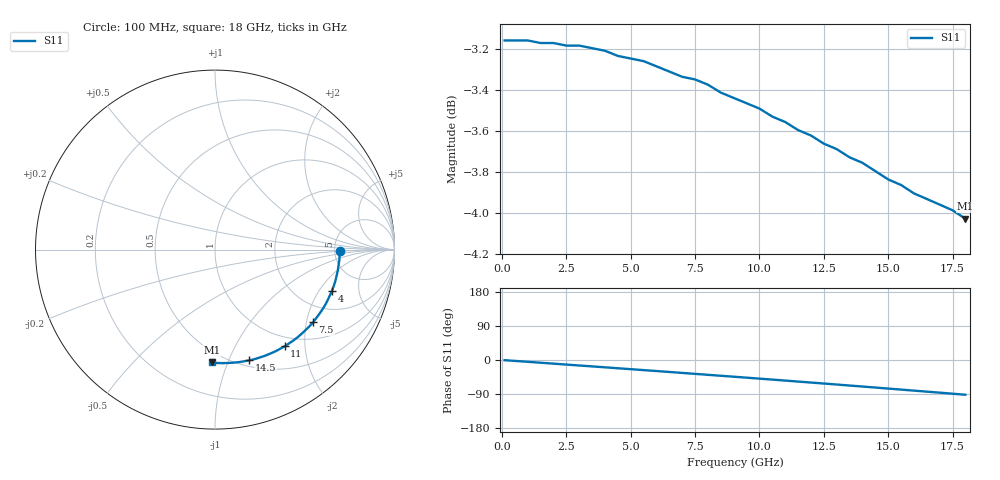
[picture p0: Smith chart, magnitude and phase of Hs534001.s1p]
!HSCH-5320 and HSCH-5340 Schottky diodes
!S-parameters at 1 mA self-bias.  Last updated 6/7/94
# ghz s ma r 50
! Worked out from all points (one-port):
!   37 points, 100 MHz to 18 GHz, reference 50 ohm
!   lowest |S11| = -4.0 dB at 18 GHz (marker M1), VSWR 4.39, Z = 21.1 - j43.9 ohm
!   |S11| at or under -10 dB: nowhere
!   S11 on the Smith chart (normalised r, x): 100 MHz: 5.55, -0.13; 4 GHz: 3.02, -2.64; 7.5 GHz: 1.45, -2.19; 11 GHz: 0.84, -1.62; 14.5 GHz: 0.56, -1.19; 18 GHz: 0.42, -0.88
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0.1  0.695 -0.5
1  0.695 -4.8
2  0.694 -9.6
2.5  0.693 -12.1
3  0.693 -14.5
4  0.691 -19.3
4.5  0.689 -21.8
5  0.688 -24.2
5.5  0.687 -26.7
6  0.685 -29.1
7  0.681 -34.1
7.5  0.68 -36.6
8  0.678 -39.1
8.5  0.675 -41.6
9.5  0.671 -46.6
10  0.669 -49.2
11  0.664 -54.3
11.5  0.661 -56.9
12  0.659 -59.5
13  0.654 -64.7
14  0.649 -70.0
14.5  0.646 -72.7
15.5  0.641 -78.1
16  0.638 -80.8
16.5  0.636 -83.5
17  0.634 -86.2
17.5  0.632 -88.9
18  0.629 -91.7
